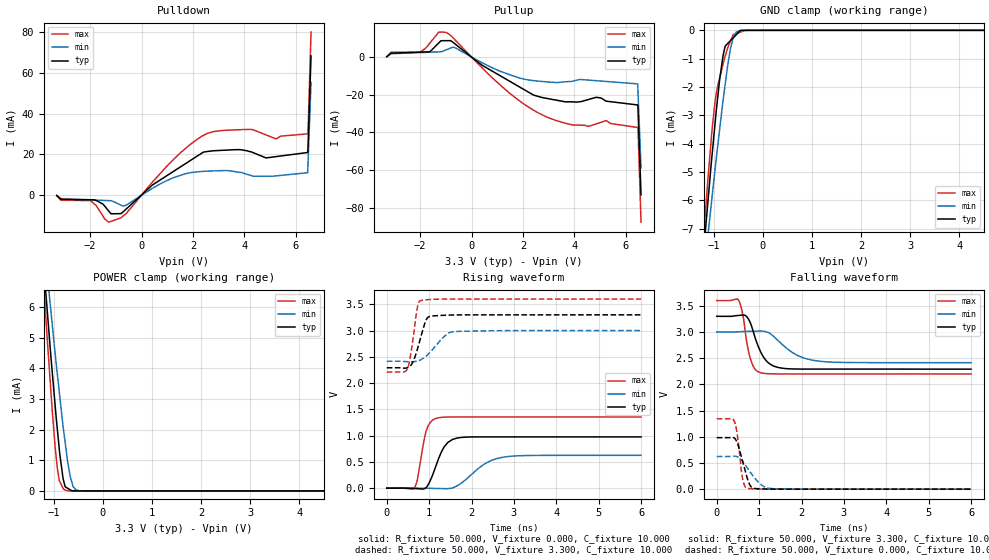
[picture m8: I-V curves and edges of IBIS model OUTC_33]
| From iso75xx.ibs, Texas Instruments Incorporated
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|   OUTC_33 MODEL
[Model]   OUTC_33
Model_type   3-state
Polarity   Non-Inverting
Vmeas = 1.65
Vref = 1.65
Cref = 15pF
Rref = 50
|   typ   min   max
| High state   (typ PVT)   (Fast PVT)  (Slow PVT)
C_comp   1.5194p   1.2464p   1.8503p
|C_comp (Low state)   1.4779p   1.2343p   1.7765p
[Voltage Range]   3.3   3.0   3.6
[Temperature Range]   27   125   -40
[Pullup Reference]   3.3   3.0   3.6
[Pulldown Reference]   -0   -0   -0
[Power Clamp Reference]   3.3   3.0   3.6
[GND Clamp Reference]   -0   -0   -0
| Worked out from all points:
|   slope of the pulldown table from 0 to 0.495 V, typ, clamps not added: 89.8 ohm
|   slope of the pullup table from 0 to 0.495 V, typ, clamps not added: 98.8 ohm
|   GND clamp passes 1 mA (typ) near -0.82 V on its own axis
|   POWER clamp passes 1 mA (typ) near -0.86 V on its own axis
|   falling waveform, R_fixture 50.000, V_fixture 3.300, C_fixture 10.000: 20-80 % time 301ps typ, 579ps min, 180ps max; typ from 3.3 V to 2.29 V
|   rising waveform, R_fixture 50.000, V_fixture 0.000, C_fixture 10.000: 20-80 % time 296ps typ, 587ps min, 183ps max; typ from -0.002 V to 0.974 V
|   rising waveform, R_fixture 50.000, V_fixture 3.300, C_fixture 10.000: 20-80 % time 220ps typ, 399ps min, 145ps max; typ from 2.29 V to 3.3 V
|   falling waveform, R_fixture 50.000, V_fixture 0.000, C_fixture 10.000: 20-80 % time 201ps typ, 352ps min, 117ps max; typ from 0.983 V to 0 V
[Pulldown]
|   Voltage   I(typ)   I(min)   I(max)
-3.3V     -220.9uA   -139.9uA   -248uA
-3.135V   -2.047mA   -1.677mA   -2.512mA
-2.002V   -2.256mA   -2.334mA   -2.632mA
-1.276V   -7.798mA   -2.689mA   -13.28mA
-665.1mV  -7.61mA    -5.273mA   -9.739mA
1.135V    10.77mA    7.992mA    16.13mA
2.567V    21.43mA    11.79mA    30.34mA
4.284V    21.19mA    9.574mA    32.27mA
5.1V      18.7mA     9.298mA    28.31mA
6.469V    20.95mA    11.01mA    30.11mA
6.481V    22.9mA     15.21mA    30.13mA
6.6V      68.36mA    55.32mA    80.06mA
[GND Clamp]
|   Voltage   I(typ)   I(min)   I(max)
-3.3V     -45.79mA   -39.57mA   -53.15mA
-1.276V   -9.163mA   -9.758mA   -8.922mA
-1.126V   -6.166mA   -7.337mA   -5.379mA
-1.056V   -4.752mA   -6.194mA   -3.905mA
-972.6mV  -3.24mA    -4.87mA    -2.485mA
-880.8mV  -1.723mA   -3.486mA   -1.677mA
-811mV    -880.4uA   -2.456mA   -1.175mA
-768.4mV  -554.6uA   -1.896mA   -907.6uA
-665.1mV  -371.7uA   -683.3uA   -392.4uA
-606.7mV  -268.2uA   -261.3uA   -160.2uA
-489.8mV  -61.18uA   -15.8uA    -79.99uA
6.6V      0A         0A         0A
[Pullup]
|   Voltage   I(typ)   I(min)   I(max)
-3.3V     214uA      144.3uA    262.4uA
-2.002V   2.612mA    2.392mA    2.626mA
-1.276V   7.498mA    2.776mA    13.23mA
-972.6mV  8.718mA    3.901mA    13.03mA
-665.1mV  7.237mA    5.099mA    9.465mA
1.273V    -11.15mA   -8.307mA   -16.73mA
2.847V    -21.75mA   -13.07mA   -31.34mA
3.98V     -23.83mA   -12.68mA   -36.17mA
5.242V    -23.42mA   -12.95mA   -33.73mA
6.469V    -25.44mA   -14.23mA   -37.4mA
6.481V    -27.41mA   -18.45mA   -37.43mA
6.6V      -73.19mA   -58.84mA   -87.72mA
[POWER Clamp]
|   Voltage   I(typ)   I(min)   I(max)
-3.3V     45.48mA    39.24mA    52.87mA
-1.276V   8.721mA    9.353mA    8.405mA
-1.126V   5.715mA    6.934mA    4.759mA
-1.056V   4.296mA    5.793mA    3.146mA
-930.9mV  2.044mA    3.839mA    759.5uA
-889.2mV  1.367mA    3.232mA    340.9uA
-811mV    394uA      2.099mA    79.98uA
-764.2mV  130.3uA    1.513mA    23.9uA
-665.1mV  35.35uA    456.5uA    2.913uA
-606.7mV  2.067uA    141.7uA    351nA
-489.8mV  1.718uA    6.206uA    110.6nA
6.6V      0A         0A         0A
[Ramp]
R_load = 50
|   typ   min   max
dV/dt_r   0.592342/2.96393e-10   0.374139/5.87144e-10   0.812425/1.83275e-10
dV/dt_f   0.621358/3.01259e-10   0.351128/5.80338e-10   0.840331/1.80404e-10
[Falling Waveform]
R_fixture = 50.000
V_fixture = 3.300
V_fixture_min = 3.000
V_fixture_max = 3.600
C_fixture = 10.000
|  time   V(typ)   V(min)   V(max)
0s        3.3V       3V         3.6V
512.3ps   3.316V     3.004V     3.613V
619.3ps   3.324V     3.009V     3.314V
709.5ps   3.291V     3.012V     2.801V
786.5ps   3.186V     3.013V     2.511V
1.016ns   2.656V     3.018V     2.227V
1.355ns   2.346V     2.906V     2.201V
1.872ns   2.294V     2.567V     2.199V
2.384ns   2.292V     2.446V     2.199V
6ns       2.291V     2.415V     2.199V
[Rising Waveform]
R_fixture = 50.000
V_fixture = 0.000
V_fixture_min = 0.000
V_fixture_max = 0.000
C_fixture = 10.000
|  time   V(typ)   V(min)   V(max)
0s        -1.699mV   2.025nV    1.597nV
643.3ps   -8.674mV   -410.2uV   -3.915mV
724.2ps   -12.25mV   -935.6uV   166mV
931.7ps   10.71mV    -3.856mV   1.09V
1.166ns   433.9mV    -7.49mV    1.328V
1.438ns   866.5mV    -10.76mV   1.353V
1.764ns   965mV      97.56mV    1.354V
2.264ns   974.3mV    435.9mV    1.354V
2.744ns   974.3mV    587.7mV    1.354V
6ns       974.2mV    623.6mV    1.354V
[Rising Waveform]
R_fixture = 50.000
V_fixture = 3.300
V_fixture_min = 3.000
V_fixture_max = 3.600
C_fixture = 10.000
|  time   V(typ)   V(min)   V(max)
0s        2.291V     2.415V     2.21V
395.5ps   2.284V     2.412V     2.209V
493.1ps   2.294V     2.407V     2.284V
566.1ps   2.336V     2.405V     2.551V
724.2ps   2.648V     2.421V     3.442V
797.3ps   2.858V     2.441V     3.57V
925.5ps   3.197V     2.511V     3.585V
984.7ps   3.259V     2.556V     3.59V
1.524ns   3.296V     2.973V     3.599V
6ns       3.3V       3V         3.6V
[Falling Waveform]
R_fixture = 50.000
V_fixture = 0.000
V_fixture_min = 0.000
V_fixture_max = 0.000
C_fixture = 10.000
|  time   V(typ)   V(min)   V(max)
0s        983.5mV    623mV      1.344V
416.6ps   973.7mV    630.9mV    1.295V
493.1ps   864.6mV    616.1mV    996.1mV
599.4ps   565.9mV    540.7mV    248.9mV
643.3ps   436.5mV    495.4mV    96.95mV
709.5ps   238.4mV    420.1mV    18.4mV
854.6ps   18.59mV    254.3mV    5.322mV
1.061ns   5.647mV    76.2mV     862uV
1.259ns   1.74mV     13.28mV    168.8uV
6ns       1.126nV    5.957nV    2.385nV
